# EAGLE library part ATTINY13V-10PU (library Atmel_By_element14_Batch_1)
8-bit Microcontroller with 1K Bytes In-System Programmable Flash
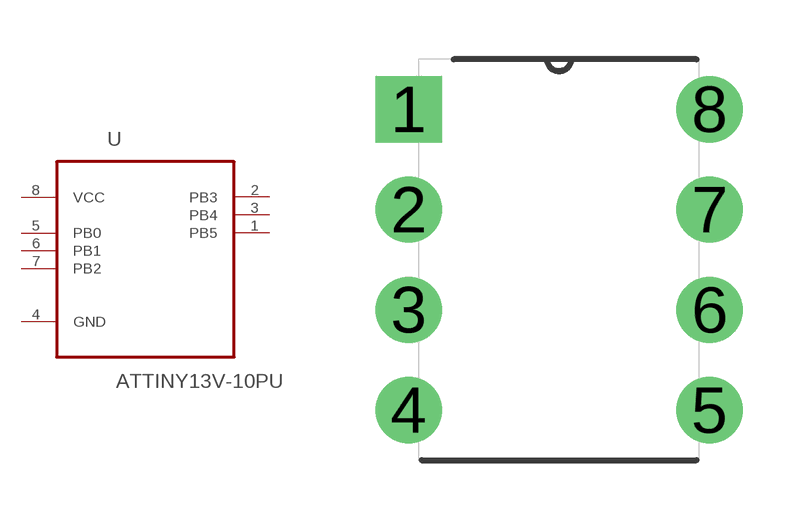
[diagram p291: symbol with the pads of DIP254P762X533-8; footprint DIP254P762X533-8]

Designator prefix U

## ATTINY13V-10PU (MPN: ATTINY13V-10PU; OC_FARNELL: 9171576; OC_NEWARK: 96K6523; PACKAGE: PDIP-8; SUPPLIER: Atmel)  [DIP254P762X533-8]
1  PB5
2  PB3
3  PB4
4  GND  pas
5  PB0
6  PB1
7  PB2
8  VCC  pwr

## Footprint DIP254P762X533-8 (pad centres in mm)
drill 1.118 square: 1 -7.62,7.62
drill 1.118: 2 -7.62,5.08; 3 -7.62,2.54; 4 -7.62,0; 5 0,0; 6 0,2.54; 7 0,5.08; 8 0,7.62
